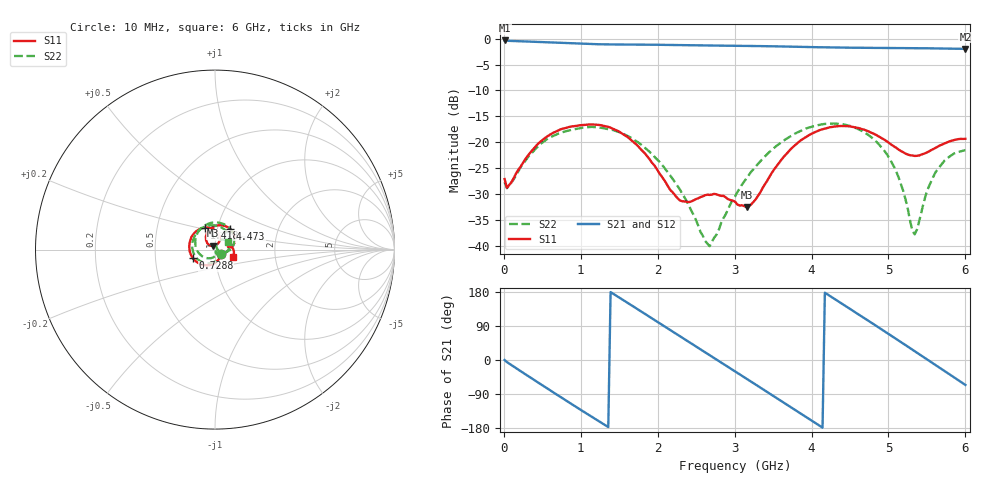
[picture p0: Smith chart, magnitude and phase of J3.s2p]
!Agilent Technologies,E8364B,MY43040528,A.07.50.67
!Agilent E8364B: A.07.50.67
!Date: Sunday, September 28, 2025 21:32:56
!Correction: S11(Full 2 Port(1,2))
!S21(Full 2 Port(1,2))
!S12(Full 2 Port(1,2))
!S22(Full 2 Port(1,2))
!S2P File: Measurements: S11, S21, S12, S22:
# Hz S  dB  R 50
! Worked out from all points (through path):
!   201 points, 10 MHz to 6 GHz, reference 50 ohm
!   highest |S21| = -0.36 dB at 10 MHz (marker M1); lowest = -2.0 dB at 6 GHz (marker M2)
!   group delay of S21, straight-line fit = 362 ps
!   lowest |S11| = -32.5 dB at 3.155 GHz (marker M3), VSWR 1.05, Z = 48.9 + j2.08 ohm
!   |S11| at or under -10 dB: start of sweep to end of sweep
!   |S22| runs from -40.0 to -16.4 dB; largest |S21 - S12| = 0.0035
!   S11 on the Smith chart (normalised r, x): 10 MHz: 1.07, -0.06; 728.8 MHz: 0.78, -0.08; 1.418 GHz: 0.87, +0.22; 4.473 GHz: 1.15, +0.27; 6 GHz: 1.22, -0.10
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1e7  -27.10 -37.7  -0.36 -0.0  -0.38 0.0  -27.67 -40.3
3.995e7  -28.76 -23.6  -0.41 -5.5  -0.41 -5.3  -28.85 -25.0
3.9935e8  -21.01 -106.8  -0.61 -53.4  -0.61 -53.4  -21.50 -115.5
7.288e8  -17.56 -158.8  -0.80 -96.6  -0.79 -96.5  -18.21 -174.3
1.0283e9  -16.68 163.3  -1.00 -135.3  -1.00 -135.2  -17.17 139.2
1.41765e9  -17.40 115.2  -1.14 175.4  -1.13 175.4  -17.63 79.7
1.6872e9  -19.97 84.9  -1.15 140.7  -1.14 140.8  -19.42 38.5
2.01665e9  -25.85 62.3  -1.19 98.1  -1.19 98.2  -23.66 -11.0
2.31615e9  -31.36 79.7  -1.26 59.4  -1.26 59.5  -29.86 -57.4
2.67555e9  -30.15 98.3  -1.34 12.9  -1.33 13.0  -40.04 -68.6
3.005e9  -31.45 100.0  -1.39 -29.8  -1.39 -29.7  -30.49 -79.7
3.15475e9  -32.49 116.4  -1.42 -49.3  -1.41 -49.2  -26.94 -103.7
3.3644e9  -28.81 139.8  -1.46 -76.7  -1.45 -76.6  -23.18 -138.8
3.57405e9  -24.04 136.7  -1.51 -104.1  -1.50 -104.0  -20.38 -172.2
4.0233e9  -18.19 99.1  -1.65 -162.8  -1.64 -162.7  -16.92 120.2
4.23295e9  -17.12 77.7  -1.71 169.8  -1.70 169.9  -16.42 90.6
4.47255e9  -16.89 53.5  -1.76 138.6  -1.75 138.6  -16.76 58.1
4.7421e9  -17.90 28.8  -1.78 103.1  -1.78 103.2  -18.62 23.0
5.01165e9  -20.17 11.3  -1.80 67.4  -1.79 67.5  -23.07 -8.7
5.3411e9  -22.63 12.6  -1.84 23.3  -1.84 23.4  -37.75 27.9
5.61065e9  -21.08 13.0  -1.90 -13.0  -1.89 -13.0  -25.81 68.1
6e9  -19.32 -21.4  -1.98 -65.8  -1.98 -65.7  -21.53 30.3
